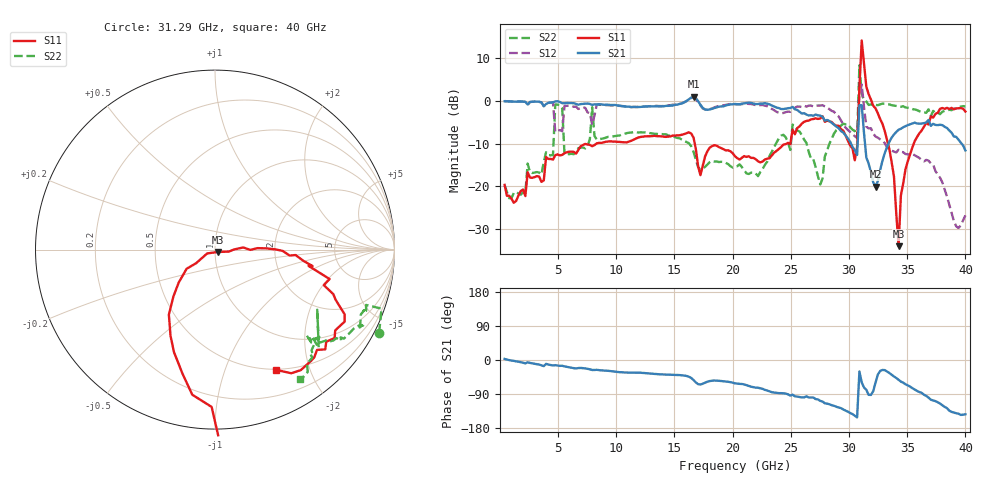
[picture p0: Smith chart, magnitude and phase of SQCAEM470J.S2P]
! Network Analyzer HP8722ES.07.66: Jul 25, 2000 Serial No. US39175408
! 27 Oct 2004  10:54:52
! Frequency  S11  S21  S12  S22
# HZ  S  DB R  50
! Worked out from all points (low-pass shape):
!   201 points, 400 MHz to 40 GHz, reference 50 ohm
!   highest |S21| = 0.99 dB at 16.64 GHz (marker M1); lowest = -20.0 dB at 32.28 GHz (marker M2)
!   |S21| within 3 dB of the highest: start of sweep to 17.62 GHz; 18 GHz to 25.4 GHz (7.408 GHz wide, 34.1 % of centre)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
!   lowest |S11| = -34.0 dB at 34.26 GHz (marker M3), VSWR 1.04, Z = 51.5 - j1.39 ohm
!   |S11| at or under -10 dB: start of sweep to 8.285 GHz; 16.74 GHz to 24.63 GHz (7.892 GHz wide, 38.1 % of centre); 33.35 GHz to 35.56 GHz (2.218 GHz wide, 6.44 % of centre)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
!   |S22| runs from -22.8 to 8.3 dB; largest |S21 - S12| = 0.95
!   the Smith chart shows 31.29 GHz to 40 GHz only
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4e8  -19.65 -91.4  -0.08 2.8  -0.02 3.6  -19.76 -87.8
4.558e9  -13.73 -117.6  -0.33 -14.5  -0.39 -15.8  -12.69 -94.4
4.756e9  -12.70 -126.3  -0.14 -13.6  -7.26 33.7  -0.83 -25.3
7.132e9  -10.32 -128.8  -0.69 -21.5  -1.48 -25.8  -10.89 -83.2
7.924e9  -10.61 -129.1  -0.93 -26.4  -5.57 12.6  -1.48 -38.6
8.32e9  -9.93 -136.2  -0.82 -25.9  -0.89 -29.3  -9.05 -98.8
1.3666e10  -8.25 -150.8  -1.31 -37.6  -1.21 -43.4  -7.80 -104.0
1.6636e10  -8.58 162.0  0.99 -52.9  0.79 -61.0  -11.91 -125.6
2.02e10  -12.95 107.5  -0.72 -61.6  -0.79 -75.9  -15.34 -66.7
2.4952e10  -10.14 41.8  -1.67 -94.0  -2.55 -117.2  -11.48 -7.7
2.515e10  -6.72 64.4  -1.39 -91.6  -2.00 -23.6  -5.54 -82.0
2.6932e10  -4.24 24.1  -3.47 -99.0  -1.34 -48.6  -13.64 -74.7
3.0694e10  -10.78 15.8  -12.65 -151.4  -8.68 -115.6  -8.71 20.4
3.0892e10  3.15 25.7  -1.03 -30.1  1.32 13.5  8.33 -86.8
3.109e10  14.13 -33.2  -1.00 -59.2  3.81 -26.0  1.58 -46.1
3.1288e10  8.64 -62.0  -7.54 -72.7  -1.50 -42.4  0.21 -26.8
3.1486e10  3.31 -64.1  -13.24 -78.6  -6.01 -51.8  -0.13 -19.5
3.2278e10  -1.74 -98.9  -20.04 -59.4  -8.33 -90.4  -0.94 -22.1
3.3466e10  -11.27 -137.8  -9.58 -34.3  -11.22 -98.7  -0.82 -27.5
3.4258e10  -33.97 -42.6  -6.74 -52.3  -11.41 -101.5  -1.34 -34.8
3.5644e10  -9.42 0.2  -5.09 -78.0  -12.72 -111.2  -2.00 -40.0
4e10  -2.48 -63.1  -11.58 -143.3  -26.78 25.1  -1.28 -56.8
